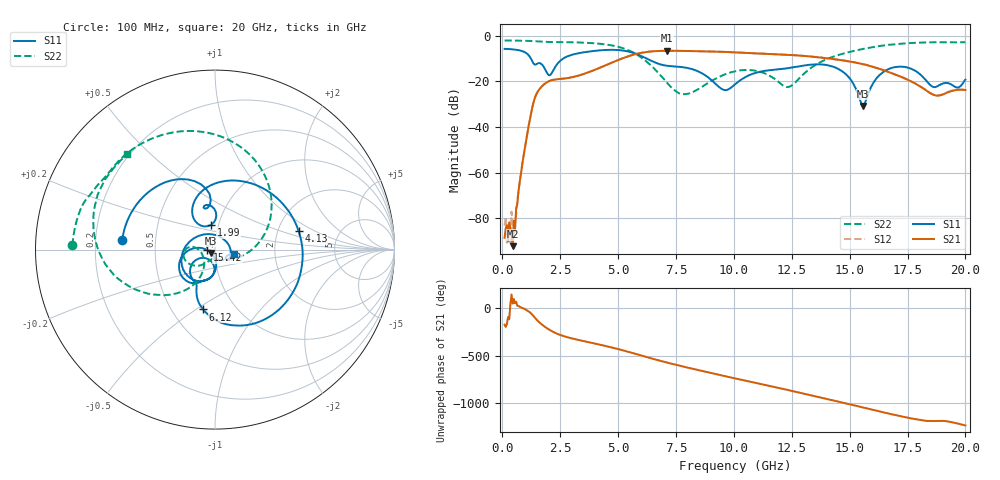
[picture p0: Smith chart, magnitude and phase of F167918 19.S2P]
!  2-Port S-parameters saved by WinCal
! VAR MeasName=S-Parameters (CALIBRATED_DATA) read from VNA (N5242A)
! VAR MeasDate=2016-11-22 10:25:41
! VAR NAME=F167918 19
! VAR FILENAME=F167918 19.S2P
! VAR DATE=2016-11-22 10:25:41
! VAR PHYS_PORTS=1,2
# Hz S DB R 50
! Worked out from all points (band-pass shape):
!   401 points, 100 MHz to 20 GHz, reference 50 ohm
!   highest |S21| = -6.53 dB at 7.115 GHz (marker M1); lowest = -92.2 dB at 448.2 MHz (marker M2)
!   |S21| within 3 dB of the highest: 5.274 GHz to 13.77 GHz (8.495 GHz wide, 89.2 % of centre)
!   lowest |S11| = -30.7 dB at 15.57 GHz (marker M3), VSWR 1.06, Z = 47.8 - j1.84 ohm
!   |S11| at or under -10 dB: 1.238 GHz to 2.621 GHz (1.383 GHz wide, 71.7 % of centre); 6.255 GHz to end of sweep
!   |S22| runs from -25.6 to -2.0 dB; largest |S21 - S12| = 0.0042
!   S11 on the Smith chart (normalised r, x): 100 MHz: 0.32, +0.05; 1.99 GHz: 0.92, +0.26; 4.13 GHz: 2.61, +0.69; 6.12 GHz: 0.71, -0.54; 15.42 GHz: 0.92, -0.01; 20 GHz: 1.24, -0.06
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1e8  -5.69 174.1  -88.57 -177.0  -83.20 -153.5  -2.00 178.3
4.4825e8  -5.90 153.1  -92.25 44.4  -82.99 70.2  -2.04 172.5
5.975e8  -6.09 143.7  -75.62 63.3  -78.73 52.2  -2.06 170.0
1.34375e9  -12.04 96.5  -29.38 -84.7  -29.36 -85.0  -2.33 157.3
1.9905e9  -17.08 98.8  -19.98 136.9  -19.95 136.7  -2.66 147.7
3.43325e9  -7.35 55.5  -16.98 15.7  -16.98 15.5  -2.93 121.2
4.12975e9  -6.43 12.4  -14.32 -21.0  -14.33 -21.0  -3.37 103.2
5.22425e9  -6.44 -55.0  -9.72 -85.6  -9.70 -85.6  -5.45 63.5
6.11975e9  -9.37 -101.1  -7.23 -146.9  -7.21 -147.1  -10.36 20.2
6.7665e9  -12.32 -115.2  -6.61 169.1  -6.59 169.1  -16.55 -15.2
7.11475e9  -13.09 -117.7  -6.53 147.0  -6.52 147.0  -20.57 -37.4
8.3585e9  -15.13 -142.0  -6.70 74.3  -6.66 74.3  -23.94 -115.3
1.005e10  -21.27 -94.9  -7.21 -18.3  -7.22 -18.2  -15.53 -153.2
1.119425e10  -15.58 -101.6  -7.77 -78.9  -7.75 -78.6  -15.95 177.9
1.23385e10  -14.16 -114.1  -8.31 -139.9  -8.28 -139.9  -22.41 -155.0
1.338325e10  -12.60 -131.3  -9.11 162.3  -9.06 162.4  -13.68 -120.0
1.467675e10  -15.52 -173.7  -10.68 89.6  -10.68 89.5  -7.91 -141.2
1.5423e10  -27.38 -176.2  -12.07 46.2  -12.08 46.2  -6.03 -153.8
1.557225e10  -30.71 -138.7  -12.38 37.7  -12.41 37.7  -5.74 -156.4
1.67165e10  -14.44 -113.0  -15.92 -28.2  -15.90 -27.7  -3.90 -177.2
1.87065e10  -22.46 44.5  -26.10 -104.1  -26.04 -103.7  -2.80 149.5
2e10  -19.19 -11.8  -23.71 -150.5  -23.59 -150.2  -2.80 132.8
